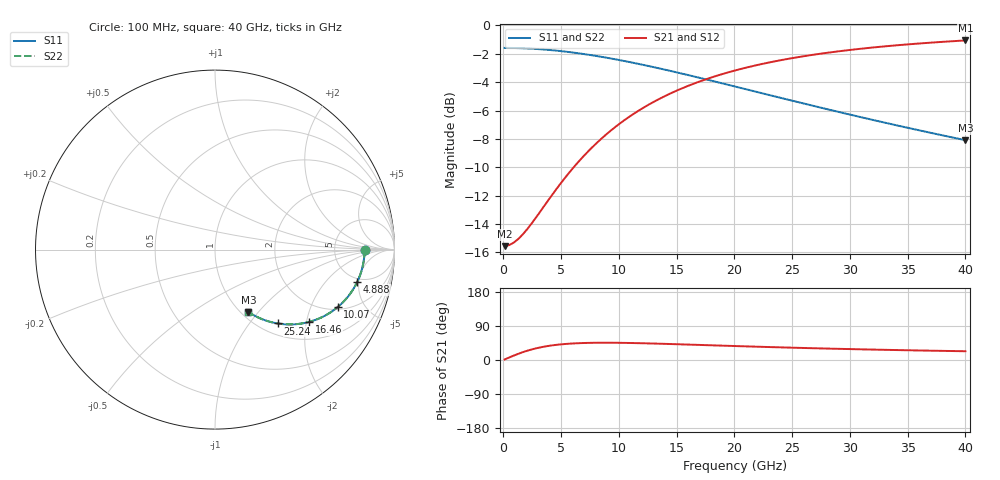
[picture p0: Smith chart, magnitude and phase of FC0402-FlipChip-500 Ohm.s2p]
!Vishay Thin-Film
!FC Family
!Case Size 0402
!Assembly Style Flip-Chip
!10/21/2015
!thinfilm@vishay.com
# GHz S MA R 50
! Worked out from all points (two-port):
!   101 points, 100 MHz to 40 GHz, reference 50 ohm
!   highest |S21| = -1.06 dB at 40 GHz (marker M1); lowest = -15.6 dB at 100 MHz (marker M2)
!   |S21| within 3 dB of the highest: 16.63 GHz to end of sweep
!   lowest |S11| = -8.1 dB at 40 GHz (marker M3), VSWR 2.30, Z = 53.9 - j44.4 ohm
!   |S11| at or under -10 dB: nowhere
!   |S22| runs from -8.1 to -1.6 dB; largest |S21 - S12| = 0
!   S11 on the Smith chart (normalised r, x): 100 MHz: 11, -0; 4.888 GHz: 4.49, -4.77; 10.07 GHz: 2.12, -3.15; 16.46 GHz: 1.45, -2.08; 25.24 GHz: 1.20, -1.39; 40 GHz: 1.08, -0.89
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0.1  0.8333 -0.3  0.1667 1.3  0.1667 1.3  0.8333 -0.3
0.499  0.8331 -1.3  0.1682 6.6  0.1682 6.6  0.8331 -1.3
0.898  0.8326 -2.4  0.1717 11.7  0.1717 11.7  0.8326 -2.4
1.696  0.8307 -4.5  0.1839 20.9  0.1839 20.9  0.8307 -4.5
2.494  0.8278 -6.6  0.2018 28.3  0.2018 28.3  0.8278 -6.6
3.292  0.8237 -8.7  0.2239 33.9  0.2239 33.9  0.8237 -8.7
4.888  0.8126 -12.8  0.2752 41.0  0.2752 41.0  0.8126 -12.8
6.085  0.8018 -15.8  0.3164 43.7  0.3164 43.7  0.8018 -15.8
6.883  0.7936 -17.8  0.3442 44.8  0.3442 44.8  0.7936 -17.8
8.479  0.7751 -21.6  0.3988 45.6  0.3988 45.6  0.7751 -21.6
10.075  0.7544 -25.2  0.451 45.3  0.451 45.3  0.7544 -25.2
11.671  0.7322 -28.5  0.4997 44.4  0.4997 44.4  0.7322 -28.5
13.666  0.703 -32.5  0.5553 42.9  0.5553 42.9  0.703 -32.5
16.459  0.6614 -37.5  0.6229 40.3  0.6229 40.3  0.6614 -37.5
20.05  0.6091 -43.1  0.6937 36.8  0.6937 36.8  0.6091 -43.1
22.444  0.5761 -46.3  0.7321 34.7  0.7321 34.7  0.5761 -46.3
25.237  0.54 -49.7  0.7697 32.3  0.7697 32.3  0.54 -49.7
26.833  0.5207 -51.4  0.7882 31.1  0.7882 31.1  0.5207 -51.4
30.025  0.4848 -54.5  0.8197 28.8  0.8197 28.8  0.4848 -54.5
33.616  0.4486 -57.5  0.848 26.5  0.848 26.5  0.4486 -57.5
36.808  0.4199 -59.8  0.8684 24.7  0.8684 24.7  0.4199 -59.8
40  0.3941 -61.9  0.8852 23.1  0.8852 23.1  0.3941 -61.9
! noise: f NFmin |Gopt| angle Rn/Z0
0.1  -1.302e-14  1  4.473e-17  9.992
4.489  3.554e-07  1  2.988e-15  3.883
8.878  1.277e-07  1  6.709e-15  1.395
13.27  -4.822e-16  1  0  0.6765
17.66  0  1  0  0.393
22.05  0  1  -1.708e-06  0.2553
26.43  1.634e-08  1  2.175e-14  0.1786
30.82  0  1  0  0.1316
35.21  0  1  -1.479e-06  0.1009
40  0  1  -1.909e-06  0.07807
